[IBIS Ver]   4.1
[File Name]   f771973xpn.ibs
[File Rev]   1.1
[Date]   DEC 06, 2019
[Source]   File originated at Texas Instruments
[Copyright]   (c) 2012, Texas Instruments Inc.
[Component]   f771973xpn
[Manufacturer] Texas Instruments
[Package]
| Variable   Typ   Min   Max
R_pkg   0.335   0.192   0.419
L_pkg   5.15E-9   4.17E-09   6.44E-09
C_pkg   5.66E-13   4.97E-13   6.69E-13
[Pin]	signal_name	model_name	R_pin	L_pin	C_pin
1	GPIO30	BCF3385DSHYPBFZ_USF	0.37739	5.941E-09	5.033E-13
2	GPIO31	BCF3385DSHYPBFZ_USF	0.36831	5.6894E-09	6.2196E-13
3	GPIO29	BCPF335585DSHYPBFZ	0.36045	5.4947E-09	6.0518E-13
4	GPIO28	BCF3385DSHYPBFZ_USF	0.34594	5.2647E-09	5.7855E-13
5	XRSN	BQ0491FS_USF	0.3377	5.0949E-09	5.6852E-13
6	GPIO46	BCF3385DSHYPBFZ_USF	0.33341	4.9689E-09	5.5261E-13
7	VDDSFL	NC	0.33211	4.8967E-09	5.3889E-13
8	VDD	NC	0.32746	4.8366E-09	5.2254E-13
9	VSS	NC	0.32958	4.8527E-09	4.9763E-13
10	A6	ICF33SHYPB_USF	0.34031	4.9415E-09	5.0964E-13
11	C6	ICF33SHYPB_USF	0.33539	4.8668E-09	5.2461E-13
12	A3	ICF33SHYPB_USF	0.32952	4.8247E-09	5.2936E-13
13	A2	ICF33SHYPB_USF	0.32918	4.8369E-09	5.3436E-13
14	A15	ICF33SHYPB_USF	0.33105	4.8874E-09	5.4006E-13
15	C4	ICF33SHYPB_USF	0.33444	4.9851E-09	5.5219E-13
16	A11	ICF33SHYPB_USF	0.34155	5.1175E-09	5.6978E-13
17	A5	ICF33SHYPB_USF	0.35186	5.2933E-09	5.8963E-13
18	A1	ICF33SHYPB_USF	0.36481	5.5182E-09	6.1125E-13
19	A0	ICF33SHYPB_USF	0.38242	5.7545E-09	6.3314E-13
20	VREFHIAC	NC	0.22218	5.2474E-09	5.7915E-13
21	VREFLOAC	NC	0.22047	5.3186E-09	5.6899E-13
22	A12	ICF33SHYPB_USF	0.37456	5.6738E-09	6.3481E-13
23	A7	ICF33SHYPB_USF	0.35627	5.4046E-09	6.0751E-13
24	A8	ICF33SHYPB_USF	0.34584	5.1698E-09	5.8725E-13
25	VSSA	NC	0.1964	4.4037E-09	6.2895E-13
26	VDDA	NC	0.19288	4.2875E-09	6.1377E-13
27	A4	ICF33SHYPB_USF	0.32817	4.7829E-09	5.3981E-13
28	C8	ICF33SHYPB_USF	0.32224	4.724E-09	5.277E-13
29	A10	ICF33SHYPB_USF	0.31894	4.6967E-09	5.0728E-13
30	VSS	NC	0.3212	4.7374E-09	4.9755E-13
31	VDD	NC	0.31999	4.7126E-09	5.0504E-13
32	VDDSFL	NC	0.33555	4.7198E-09	5.7462E-13
33	FLT2	NC	0.31808	4.726E-09	5.1417E-13
34	FLT1	NC	0.32011	4.781E-09	5.1451E-13
35	GPIO13	BCF3385DSHYPBFZ_USF	0.32052	4.8256E-09	5.3241E-13
36	GPIO12	BCF3385DSHYPBFZ_USF	0.32254	4.9253E-09	5.4909E-13
37	GPIO11	BCF3385DSHYPBFZ_USF	0.3265	5.058E-09	5.579E-13
38	GPIO33	BCPF335585DSHYPBFZ	0.35174	5.4283E-09	5.8845E-13
39	GPIO16	BCF3385DSHYPBFZ_USF	0.37868	5.8223E-09	6.3024E-13
40	GPIO17	BCF3385DSHYPBFZ_USF	0.4044	6.241E-09	5.3603E-13
41	GPIO24	BCPF335585DSHYPBFZ	0.41093	6.2936E-09	5.3069E-13
42	GPIO25	BCF3385DSHYPBFZ_USF	0.38799	5.9093E-09	6.3422E-13
43	GPIO26	BCF3385DSHYPBFZ_USF	0.37158	5.6306E-09	6.1091E-13
44	GPIO27	BCF3385DSHYPBFZ_USF	0.36124	5.4296E-09	5.9097E-13
45	TCK	BCF3355DSHYPBFZ_TMS_USF	0.35009	5.2218E-09	5.7901E-13
46	TDO_GPIO37	BCPF335585DSHYPBFZ	0.35092	5.113E-09	5.6245E-13
47	TMS	BCF3355DSHYPBFZ_TMS_USF	0.3353	4.9307E-09	5.4119E-13
48	TDI_GPIO35	BCF3385DSHYPBFZ_USF	0.33203	4.8438E-09	5.3552E-13
49	GPIO32	BCPF335585DSHYPBFZ	0.34221	4.8647E-09	5.3557E-13
50	GPIO18_X2	BCPF335585DSHYPBFZ	0.1968	4.2235E-09	5.898E-13
51	GPIO19_X1	BCF3385DSHYPBFZ_USF	0.19716	4.1792E-09	5.8792E-13
52	VDDSFL	NC	0.32039	4.7721E-09	6.5156E-13
53	VDD	NC	0.31105	4.8092E-09	6.693E-13
54	GPIO43	BCF3385DSHYPBFZ_USF	0.32709	4.8689E-09	5.4758E-13
55	VSS_VREGENZ	NC	0.31548	4.924E-09	5.9399E-13
56	GPIO39	BCF3385DSHYPBFZ_USF	0.32906	5.0302E-09	5.4388E-13
57	GPIO42	BCF3385DSHYPBFZ_USF	0.33094	5.1084E-09	5.5861E-13
58	GPIO8	BCF3385DSHYPBFZ_USF	0.35263	5.4516E-09	5.9659E-13
59	GPIO4	BCF3385DSHYPBFZ_USF	0.38185	5.8506E-09	6.2568E-13
60	GPIO3	BCF3385DSHYPBFZ_USF	0.4197	6.4447E-09	5.3218E-13
61	GPIO2	BCF3385DSHYPBFZ_USF	0.41623	6.3365E-09	5.3541E-13
62	GPIO1	BCPF335585DSHYPBFZ	0.40426	6.0571E-09	6.3936E-13
63	GPIO0	BCF3385DSHYPBFZ_USF	0.37654	5.7104E-09	6.054E-13
64	GPIO40	BCF3385DSHYPBFZ_USF	0.37672	5.6348E-09	5.9668E-13
65	GPIO23	BCF3385DSHYPBFZ_USF	0.36399	5.3682E-09	5.8852E-13
66	GPIO41	BCF3385DSHYPBFZ_USF	0.34945	5.1547E-09	5.6708E-13
67	GPIO22	BCF3385DSHYPBFZ_USF	0.33966	4.9779E-09	5.4842E-13
68	GPIO7	BCF3385DSHYPBFZ_USF	0.32994	4.8292E-09	5.3659E-13
69	GPIO44	BCF3385DSHYPBFZ_USF	0.32532	4.7499E-09	5.2633E-13
70	VSS	NC	0.32114	4.7087E-09	5.1678E-13
71	VDD	NC	0.32513	4.7661E-09	6.0366E-13
72	VDDSFL_VDDSFL_SENSE	NC	0.30543	4.6459E-09	5.7078E-13
73	GPIO45	BCF3385DSHYPBFZ_USF	0.32107	4.6979E-09	5.2972E-13
74	GPIO5	BCF3385DSHYPBFZ_USF	0.32109	4.7501E-09	5.3518E-13
75	GPIO9	BCF3385DSHYPBFZ_USF	0.32372	4.8488E-09	5.4775E-13
76	GPIO10	BCF3385DSHYPBFZ_USF	0.33027	4.9917E-09	5.6466E-13
77	GPIO34	BCF3385DSHYPBFZ_USF	0.34014	5.1738E-09	5.8444E-13
78	GPIO15	BCF3385DSHYPBFZ_USF	0.35218	5.4037E-09	5.9832E-13
79	GPIO14	BCF3385DSHYPBFZ_USF	0.36796	5.6465E-09	6.0686E-13
80	GPIO6	BCF3385DSHYPBFZ_USF	0.37888	5.9441E-09	5.025E-13
| End of package information
|   Component IQ0440FS_VREGENZ_USF
[Component]   IQ0440FS_VREGENZ_USF
[Manufacturer]   Texas Instruments
[Package]
|  variable   typ   min   max
R_pkg   0   0   0
L_pkg   0   0   0
C_pkg   0   0   0
[Pin]   signal_name   model_name   R_pin   L_pin   C_pin
VSS   VSS   GND
VDDS   VDDS   POWER
PAD   PAD   IQ0440FS_VREGENZ_USF
[Model Selector] IQ0440FS_VREGENZ_USF
VREGENZ_WK_PD_ON_3P3  Cell operated at 3.3(nom)
|VREGENZ_WK_PD_ON_3P3; WEAK_PULLDOWN_ON
VREGENZ_WK_PD_OFF_3P3  Cell operated at 3.3(nom)
|   Component ICF33SHYPB_USF
[Component]   ICF33SHYPB_USF
[Manufacturer]   Texas Instruments
[Package]
|  variable   typ   min   max
R_pkg   0   0   0
L_pkg   0   0   0
C_pkg   0   0   0
[Pin]   signal_name   model_name   R_pin   L_pin   C_pin
VSS   VSS   GND
VDDS   VDDS   POWER
PAD   PAD   ICF33SHYPB_USF
[Model Selector] ICF33SHYPB_USF
ICF_WK_PUPD_OFF_3P3  Cell operated at 3.3(nom)
|ICF_WK_PUPD_OFF_3P3; WEAK_PULL_OFF
ICF_WK_PU_ON_3P3  Cell operated at 3.3(nom)
|ICF_WK_PU_ON_3P3; WEAK_PULLUP_ON
ICF_WK_PD_ON_3P3  Cell operated at 3.3(nom)
|   Component ICF33SHYPB_FS_SFII_CUS
[Component]   ICF33SHYPB_FS_SFII_CUS
[Manufacturer]   Texas Instruments
[Package]
|  variable   typ   min   max
R_pkg   0   0   0
L_pkg   0   0   0
C_pkg   0   0   0
[Pin]   signal_name   model_name   R_pin   L_pin   C_pin
VSS   VSS   GND
VDDS   VDDS   POWER
PAD   PAD   ICF33SHYPB_FS_SFII_CUS
[Model Selector] ICF33SHYPB_FS_SFII_CUS
CUS_WK_PUPD_OFF_3P3  Cell operated at 3.3(nom)
|CUS_WK_PUPD_OFF_3P3; WEAK_PULL_OFF
CUS_WK_PU_ON_3P3  Cell operated at 3.3(nom)
|CUS_WK_PU_ON_3P3; WEAK_PULLUP_ON
CUS_WK_PD_ON_3P3  Cell operated at 3.3(nom)
|   Component BT3308BT5FSHYPB_SFII
[Component]   BT3308BT5FSHYPB_SFII
[Manufacturer]   Texas Instruments
[Package]
|  variable   typ   min   max
R_pkg   0   0   0
L_pkg   0   0   0
C_pkg   0   0   0
[Pin]   signal_name   model_name   R_pin   L_pin   C_pin
VSS   VSS   GND
VDDS   VDDS   POWER
PAD   PAD   BT3308BT5FSHYPB_SFII
[Model Selector] BT3308BT5FSHYPB_SFII
BT_OPEN_DRAIN_6MA_3P3  Cell operated at 3.3(nom)
|BT_OPEN_DRAIN_6MA_3P3
BT_WEAK_PD_ON_3P3  Cell operated at 3.3(nom)
|BT_WEAK_PD_ON_3P3
BT_OPEN_DRAIN_3MA_3P3  Cell operated at 3.3(nom)
|BT_OPEN_DRAIN_3MA_3P3
BT_DRIVER_MODE_6MA_3P3  Cell operated at 3.3(nom)
|BT_DRIVER_MODE_6MA_3P3
BT_DRIVER_MODE_3MA_3P3  Cell operated at 3.3(nom)
|BT_DRIVER_MODE_3MA_3P3
BT_WEAK_PU_ON_3P3  Cell operated at 3.3(nom)
|   Component BQ0491FS_USF
[Component]   BQ0491FS_USF
[Manufacturer]   Texas Instruments
[Package]
|  variable   typ   min   max
R_pkg   0   0   0
L_pkg   0   0   0
C_pkg   0   0   0
[Pin]   signal_name   model_name   R_pin   L_pin   C_pin
VSS   VSS   GND
VDDS   VDDS   POWER
PAD   PAD   BQ0491FS_USF
[Model Selector] BQ0491FS_USF
XRSN_WK_PU_ON_3P3  Cell operated at 3.3(nom)
|XRSN_WK_PU_ON_3P3; WEAK_PULLUP_ON
XRSN_OPEN_DRAIN  Cell operated at 3.3(nom)
|   Component BCPF335585DSHYPBFZ
[Component]   BCPF335585DSHYPBFZ
[Manufacturer]   Texas Instruments
[Package]
|  variable   typ   min   max
R_pkg   0   0   0
L_pkg   0   0   0
C_pkg   0   0   0
[Pin]   signal_name   model_name   R_pin   L_pin   C_pin
VSS   VSS   GND
VDDS   VDDS   POWER
PAD   PAD   BCPF335585DSHYPBFZ
[Model Selector] BCPF335585DSHYPBFZ
BCPF_WK_PU_ON_3P3  Cell operated at 3.3(nom)
|BCPF_WK_PU_ON_3P3; WEAK_PULLUP_ON
BCPF_DRIVER_4MA_3P3  Cell operated at 3.3(nom)
|BCPF_DRIVER_4MA_3P3
BCPF_DRIVER_2MA_3P3  Cell operated at 3.3(nom)
|BCPF_DRIVER_2MA_3P3
BCPF_WK_PD_ON_3P3  Cell operated at 3.3(nom)
|   Component BCF3385DSHYPBFZ_USF
[Component]   BCF3385DSHYPBFZ_USF
[Manufacturer]   Texas Instruments
[Package]
|  variable   typ   min   max
R_pkg   0   0   0
L_pkg   0   0   0
C_pkg   0   0   0
[Pin]   signal_name   model_name   R_pin   L_pin   C_pin
VSS   VSS   GND
VDDS   VDDS   POWER
PAD   PAD   BCF3385DSHYPBFZ_USF
[Model Selector] BCF3385DSHYPBFZ_USF
BCF3385DUSF_WK_PU  Cell operated at 3.3(nom)
| BCF3385DUSF_WK_PU; WEAK_PULLUP_ON
BCF3385DUSF_DRIVER_3P3  Cell operated at 3.3(nom)
|BCF3385DUSF_DRIVER_3P3
BCF3385DUSF_WK_PD  Cell operated at 3.3(nom)
|   Component BCF3385DSHYPBFZ
[Component]   BCF3385DSHYPBFZ
[Manufacturer]   Texas Instruments
[Package]
|  variable   typ   min   max
R_pkg   0   0   0
L_pkg   0   0   0
C_pkg   0   0   0
[Pin]   signal_name   model_name   R_pin   L_pin   C_pin
VSS   VSS   GND
VDDS   VDDS   POWER
PAD   PAD   BCF3385DSHYPBFZ
[Model Selector] BCF3385DSHYPBFZ
BCF3385D_WK_PU_3P3  Cell operated at 3.3(nom)
|BCF3385D_WK_PU_3P3; WEAK_PULLUP_ON
BCF3385D_DRIVER_3P3  Cell operated at 3.3(nom)
|BCF3385D_DRIVER_3P3
BCF3385D_WK_PD_3P3  Cell operated at 3.3(nom)
|   Component BCF3355DSHYPBFZ_TMS_USF
[Component]   BCF3355DSHYPBFZ_TMS_USF
[Manufacturer]   Texas Instruments
[Package]
|  variable   typ   min   max
R_pkg   0   0   0
L_pkg   0   0   0
C_pkg   0   0   0
[Pin]   signal_name   model_name   R_pin   L_pin   C_pin
VSS   VSS   GND
VDDS   VDDS   POWER
PAD   PAD   BCF3355DSHYPBFZ_TMS_USF
[Model Selector] BCF3355DSHYPBFZ_TMS_USF
TMS_WK_PU_ON_3P3  Cell operated at 3.3(nom)
|TMS_WK_PU_ON_3P3; WEAK_PULLUP_ON
TMS_DRIVER_3P3  Cell operated at 3.3(nom)
|TMS_DRIVER_3P3
TMS_WK_PD_ON_3P3  Cell operated at 3.3(nom)
|   Component BCF3335DSHYPBFZ
[Component]   BCF3335DSHYPBFZ
[Manufacturer]   Texas Instruments
[Package]
|  variable   typ   min   max
R_pkg   0   0   0
L_pkg   0   0   0
C_pkg   0   0   0
[Pin]   signal_name   model_name   R_pin   L_pin   C_pin
VSS   VSS   GND
VDDS   VDDS   POWER
PAD   PAD   BCF3335DSHYPBFZ
[Model Selector] BCF3335DSHYPBFZ
BCF3335D_WK_PU_3P3  Cell operated at 3.3(nom)
|BCF3335D_WK_PU_3P3; WEAK_PULLUP_ON
BCF3335D_DRIVER_3P3  Cell operated at 3.3(nom)
|BCF3335D_DRIVER_3P3
BCF3335D_WK_PD_3P3  Cell operated at 3.3(nom)
| Models and submodels in the file (32): VREGENZ_WK_PD_ON_3P3 (Input), VREGENZ_WK_PD_OFF_3P3 (Input), ICF_WK_PUPD_OFF_3P3 (Input), ICF_WK_PU_ON_3P3 (Input), ICF_WK_PD_ON_3P3 (Input), CUS_WK_PUPD_OFF_3P3 (Input), CUS_WK_PU_ON_3P3 (Input), CUS_WK_PD_ON_3P3 (Input), BT_OPEN_DRAIN_6MA_3P3 (I/O_open_drain), BT_WEAK_PD_ON_3P3 (Input), BT_OPEN_DRAIN_3MA_3P3 (I/O_open_drain), BT_DRIVER_MODE_6MA_3P3 (I/O), BT_DRIVER_MODE_3MA_3P3 (I/O), BT_WEAK_PU_ON_3P3 (Input), XRSN_WK_PU_ON_3P3 (Input), XRSN_OPEN_DRAIN (I/O_open_drain), BCPF_WK_PU_ON_3P3 (Input), BCPF_DRIVER_4MA_3P3 (I/O), BCPF_DRIVER_2MA_3P3 (I/O), BCPF_WK_PD_ON_3P3 (Input), BCF3385DUSF_WK_PU (Input), BCF3385DUSF_DRIVER_3P3 (I/O), BCF3385DUSF_WK_PD (Input), BCF3385D_WK_PU_3P3 (Input), BCF3385D_DRIVER_3P3 (I/O), BCF3385D_WK_PD_3P3 (Input), TMS_WK_PU_ON_3P3 (Input), TMS_DRIVER_3P3 (I/O), TMS_WK_PD_ON_3P3 (Input), BCF3335D_WK_PU_3P3 (Input), BCF3335D_DRIVER_3P3 (I/O), BCF3335D_WK_PD_3P3 (Input)
